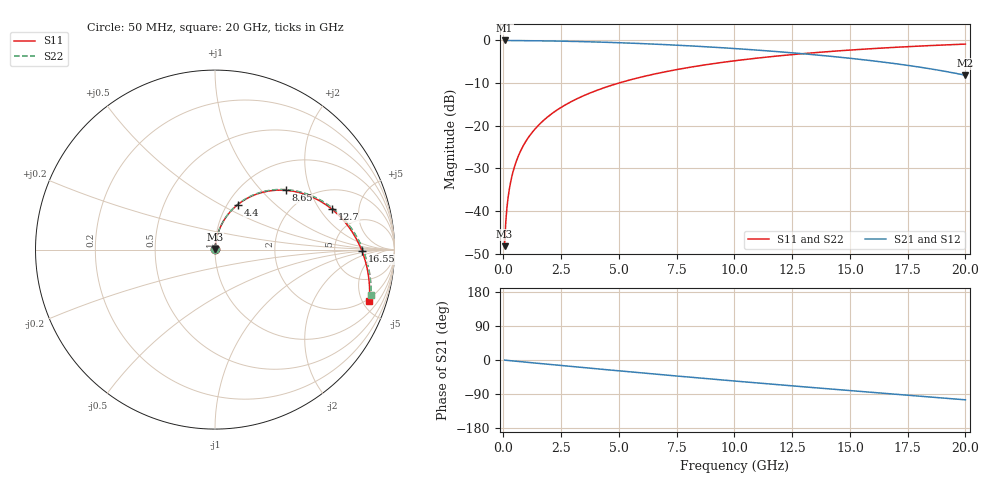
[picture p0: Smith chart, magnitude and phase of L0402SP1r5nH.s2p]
!	AVX Thin Film Operation
!	Date:		5 January 2004
!	Description: 	Accu-L®  L0402 Series Thin Film RF Inductors
!	Part Number:	L04021R5AHLTR
!	50 MHz-20GHz Serial Measurements
#	mhz	S	db	R	50
!	S11	S11	S21	S21	S12	S12	S22	S22
!	dB	Phase	dB	Phase	dB	Phase	dB	Phase
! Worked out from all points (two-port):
!   400 points, 50 MHz to 20 GHz, reference 50 ohm
!   highest |S21| = 0.00 dB at 50 MHz (marker M1); lowest = -8.2 dB at 20 GHz (marker M2)
!   |S21| within 3 dB of the highest: start of sweep to 12.72 GHz
!   lowest |S11| = -48.2 dB at 50 MHz (marker M3), VSWR 1.01, Z = 50 + j0.385 ohm
!   |S11| at or under -10 dB: start of sweep to 4.989 GHz
!   |S22| runs from -48.2 to -0.9 dB; largest |S21 - S12| = 2
!   S11 on the Smith chart (normalised r, x): 50 MHz: 1.00, +0.01; 4.4 GHz: 1.12, +0.61; 8.65 GHz: 1.54, +1.38; 12.7 GHz: 3.06, +2.62; 16.55 GHz: 10, -0; 20 GHz: 1.80, -5.67
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50  -48.23 82.6  -0.00 -0.3  -0.00 179.7  -48.23 82.6
100  -42.59 83.8  -0.01 -0.6  -0.01 179.4  -42.59 83.8
150  -39.25 84.2  -0.01 -0.9  -0.01 179.1  -39.25 84.2
250  -35.01 84.4  -0.01 -1.5  -0.01 178.5  -35.01 84.4
350  -32.21 84.3  -0.02 -2.1  -0.02 177.9  -32.21 84.3
450  -30.10 84.0  -0.02 -2.7  -0.02 177.3  -30.10 84.0
600  -27.69 83.4  -0.03 -3.6  -0.03 176.4  -27.69 83.4
800  -25.27 82.5  -0.04 -4.7  -0.04 175.3  -25.27 82.6
1250  -21.51 80.3  -0.06 -7.3  -0.06 172.7  -21.51 80.4
1800  -18.44 77.4  -0.10 -10.5  -0.10 169.5  -18.44 77.5
2500  -15.68 73.6  -0.17 -14.5  -0.17 165.5  -15.68 73.7
3400  -13.13 68.6  -0.27 -19.6  -0.27 160.4  -13.13 68.8
4400  -11.01 63.1  -0.43 -25.2  -0.43 154.8  -11.01 63.4
6700  -7.69 50.5  -0.90 -37.9  -0.90 142.1  -7.69 51.0
8650  -5.79 40.0  -1.45 -48.4  -1.45 131.6  -5.79 40.7
10050  -4.74 32.7  -1.91 -55.7  -1.91 124.3  -4.74 33.4
12700  -3.22 19.0  -2.99 -69.3  -2.99 110.7  -3.22 20.0
13350  -2.92 15.6  -3.30 -72.5  -3.30 107.5  -2.92 16.7
16550  -1.74 -0.5  -5.15 -88.3  -5.15 91.7  -1.73 0.9
16700  -1.69 -1.3  -5.26 -89.0  -5.26 91.0  -1.69 0.2
18400  -1.22 -9.9  -6.58 -97.3  -6.58 82.7  -1.22 -8.2
20000  -0.86 -18.2  -8.16 -105.1  -8.16 74.9  -0.86 -16.2
